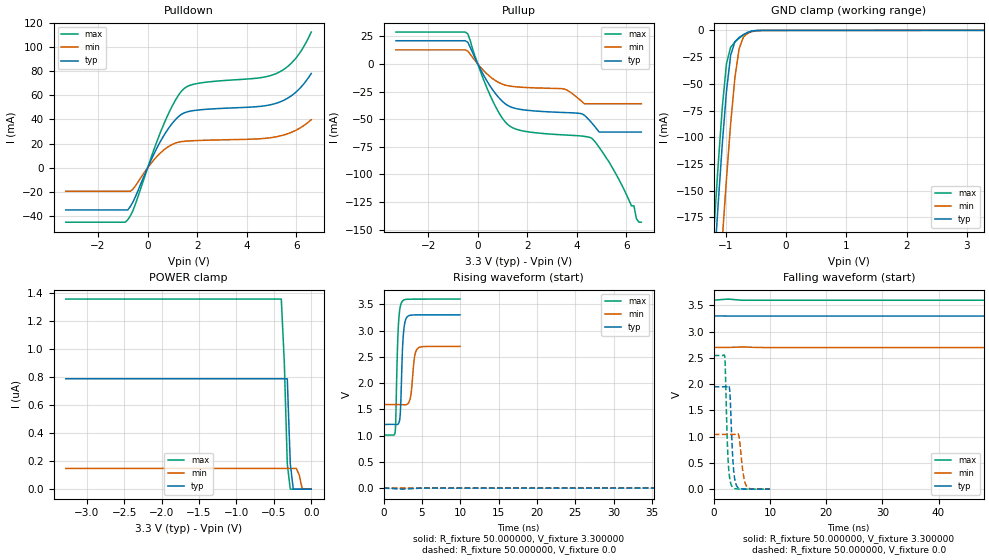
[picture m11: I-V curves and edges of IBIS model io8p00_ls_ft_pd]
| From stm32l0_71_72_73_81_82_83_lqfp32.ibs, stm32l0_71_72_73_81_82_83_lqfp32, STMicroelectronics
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|   Model io8p00_ls_ft_pd
[Model]  io8p00_ls_ft_pd
Model_type I/O
Polarity   Non-Inverting
Enable   Active-Low
Vinl =   0.990000V
Vinh =   2.310000V
Vmeas =  1.650000V
Cref =   50.000000pF
Rref =   100.000000M
Vref =   0.0V
C_comp   4.606100pF   4.563500pF   4.706200pF
[Temperature Range]   25.000000   0.125000k   -40.000000
[Pullup Reference]   3.300000V   2.700000V   3.600000V
[Pulldown Reference]   0.0V   0.0V   0.0V
[POWER Clamp Reference]   3.300000V   2.700000V   3.600000V
[GND Clamp Reference]   0.0V   0.0V   0.0V
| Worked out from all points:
|   slope of the pulldown table from 0 to 0.495 V, typ, clamps not added: 23.6 ohm
|   slope of the pullup table from 0 to 0.495 V, typ, clamps not added: 24.9 ohm
|   GND clamp passes 1 mA (typ) near -0.59 V on its own axis
|   rising waveform, R_fixture 50.000000, V_fixture 3.300000: 20-80 % time 316ps typ, 427ps min, 299ps max; typ from 1.21 V to 3.3 V
|   rising waveform, R_fixture 50.000000, V_fixture 0.0: 20-80 % time 204ns typ, 424ns min, 100ns max; typ from 0 V to 1.95 V
|   falling waveform, R_fixture 50.000000, V_fixture 3.300000: 20-80 % time 194ns typ, 380ns min, 107ns max; typ from 3.3 V to 1.21 V
|   falling waveform, R_fixture 50.000000, V_fixture 0.0: 20-80 % time 519ps typ, 682ps min, 457ps max; typ from 1.95 V to 0 V
[Pulldown]
|Voltage   I(typ)   I(min)   I(max)
-3.3V     -34.78mA   -19.34mA   -44.89mA
-900mV    -34.78mA   -19.34mA   -44.89mA
-800mV    -34.78mA   -19.34mA   -42.84mA
-600mV    -28.56mA   -17.8mA    -35.74mA
100mV     4.638mA    2.744mA    6.076mA
600mV     24.8mA     13.84mA    33.52mA
1V        36.92mA    19.39mA    51.35mA
1.4V      44.67mA    21.76mA    64.17mA
2V        47.7mA     22.58mA    69.7mA
5.2V      53.44mA    25.71mA    78.04mA
6V        62.89mA    31.28mA    91.14mA
6.6V      77.95mA    39.75mA    112.2mA
[Pullup]
|Voltage   I(typ)   I(min)   I(max)
-3.3V     21.04mA    12.78mA    28.86mA
-400mV    19.64mA    11.53mA    27.22mA
400mV     -16.48mA   -9.566mA   -23.24mA
1.1V      -35.89mA   -19.06mA   -52.22mA
1.7V      -41.02mA   -20.95mA   -60.01mA
3.5V      -43.95mA   -22.7mA    -64.24mA
4.2V      -45.08mA   -33.97mA   -65.24mA
4.6V      -53.38mA   -35.99mA   -67.23mA
4.9V      -61.64mA   -35.99mA   -75.5mA
6.3V      -61.64mA   -35.99mA   -128.4mA
6.4V      -61.64mA   -35.99mA   -140mA
6.6V      -61.64mA   -35.99mA   -143.2mA
[GND_clamp]
|Voltage   I(typ)   I(min)   I(max)
-3.3V     -2.276A    -2.356A    -2.25A
-1.2V     -226mA     -318.7mA   -189.2mA
-1.13V    -164.9mA   -256.6mA   -128.3mA
-1.06V    -107.5mA   -196.5mA   -72.79mA
-990mV    -57.33mA   -139.4mA   -31.4mA
-920mV    -23.23mA   -87.33mA   -15.73mA
-850mV    -10.59mA   -44.46mA   -10.94mA
-780mV    -6.551mA   -17.26mA   -7.364mA
-710mV    -3.945mA   -6.365mA   -4.316mA
-640mV    -1.966mA   -2.806mA   -1.983mA
-360mV    -10.16uA   -28.12uA   -6.105uA
3.28V     73.92uA    88.6uA     51.45uA
[POWER_clamp]
|Voltage   I(typ)   I(min)   I(max)
-3.28V    786.7nA    148nA      1.355uA
-400mV    786.7nA    148nA      1.355uA
-360mV    786.7nA    148nA      908.2nA
-320mV    786.7nA    148nA      180.5nA
-280mV    182.6nA    148nA      0A
-240mV    0A         148nA      0A
-200mV    0A         148nA      0A
-160mV    0A         101.6nA    0A
-120mV    0A         0A         0A
0V        0A         0A         0A
[Ramp]
| variable   typ   min   max
dV/dt_r  1.17009/0.20418u   0.60143/0.42574u   1.52718/0.10003u
dV/dt_f  1.25010/0.19406u   0.62496/0.38061u   1.55262/0.10676u
R_load = 50.000000
[Rising Waveform]
R_fixture= 50.000000
V_fixture= 3.300000
V_fixture_min= 2.700000
V_fixture_max= 3.600000
|time   V(typ)   V(min)   V(max)
0s        1.213V     1.591V     1.011V
1.502ns   1.212V     1.591V     1.067V
1.902ns   1.222V     1.591V     3.035V
2.162ns   1.407V     1.591V     3.447V
2.362ns   2.236V     1.589V     3.54V
2.643ns   3.031V     1.586V     3.581V
3.103ns   3.265V     1.6V       3.595V
3.524ns   3.291V     1.747V     3.596V
4.404ns   3.297V     2.655V     3.597V
9.97ns    3.298V     2.698V     3.599V
[Rising Waveform]
R_fixture= 50.000000
V_fixture= 0.0
V_fixture_min= 0.0
V_fixture_max= 0.0
|time   V(typ)   V(min)   V(max)
0s        47.9uV     15.55uV    94.68uV
50.05ns   966.7uV    -22.39uV   85.3mV
100.1ns   73.78mV    11.25uV    897.7mV
160.2ns   413.3mV    5.894mV    1.837V
200.2ns   698.2mV    12.67mV    2.212V
247.7ns   1.023V     46.24mV    2.419V
355.4ns   1.543V     182.6mV    2.524V
508ns     1.844V     443.7mV    2.543V
855.9ns   1.946V     885.4mV    2.545V
1.246us   1.95V      1.042V     2.545V
[Falling Waveform]
R_fixture= 50.000000
V_fixture= 3.300000
V_fixture_min= 2.700000
V_fixture_max= 3.600000
|time   V(typ)   V(min)   V(max)
0s        3.298V     2.698V     3.599V
82.58ns   3.296V     2.695V     3.496V
145.1ns   3.211V     2.695V     2.607V
215.2ns   2.837V     2.692V     1.61V
255.3ns   2.567V     2.68V      1.247V
292.8ns   2.305V     2.657V     1.117V
407.9ns   1.604V     2.529V     1.037V
520.5ns   1.347V     2.338V     1.019V
845.8ns   1.23V      1.786V     1.011V
1.246us   1.213V     1.591V     1.011V
[Falling Waveform]
R_fixture= 50.000000
V_fixture= 0.0
V_fixture_min= 0.0
V_fixture_max= 0.0
|time   V(typ)   V(min)   V(max)
0s        1.95V      1.042V     2.545V
1.942ns   1.95V      1.042V     2.526V
2.042ns   1.95V      1.042V     2.343V
2.523ns   1.962V     1.042V     611.5mV
2.843ns   1.869V     1.042V     201.9mV
3.123ns   1.173V     1.042V     77.46mV
3.544ns   350.4mV    1.042V     19.08mV
4.144ns   49.96mV    1.063V     3.716mV
5.806ns   789.5uV    60.11mV    926.9uV
9.97ns    47.9uV     15.55uV    94.68uV
